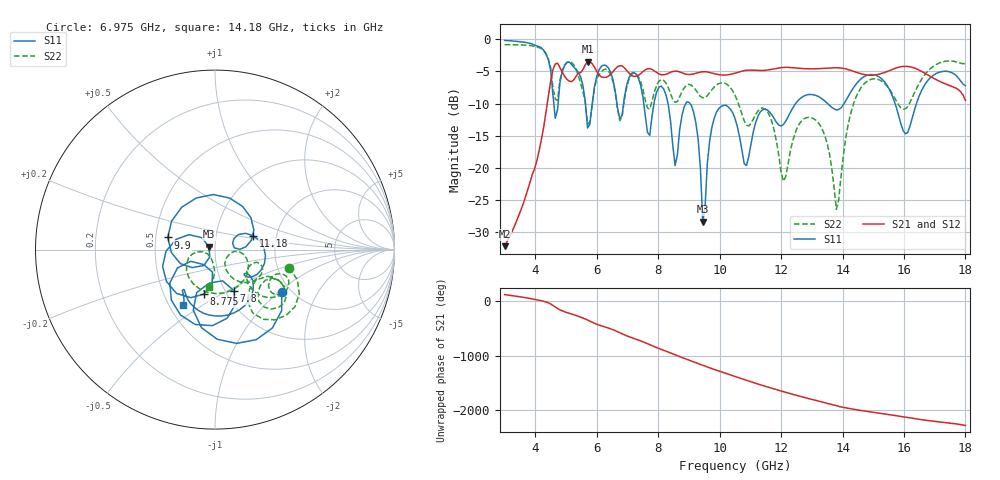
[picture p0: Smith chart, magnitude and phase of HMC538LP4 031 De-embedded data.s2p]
! Chelmsford, MA 01824
! http://www.hittite.com
! Tel: 978-250-3343
! Fax: 978-250-3373
! Device  :  HMC538LP4
! Description:  600 Analog Phase Shifter
! Frequency  :  6.0 GHz - 15.0 GHz
! Package  :  LP4  - 4x4 mm Quad Flatpack No-Lead (QFN) Plastic Package: 24 pin
! Ports  :  2 RF, 1 DC
!  Pin  3  = Rfin  = Port 1
!  Pin  16  = Rfout = Port 2
!  pin  21  = vCTL
! Voltages:  VCTL  = 0 to 5.0 Volts
! Currents :  Vb(V)  Vd(V)  Ib(mA)  Id(mA)
!  0.00  3.10  0.000000	0.467830
! Data:  The device was measured on evaluation board 111296-1.
!  Data was collected using a calibrated network analyzer.
!  The evaluation circuit board was modeled and simulated.This was use
!  to removed the evaluation board circuit from the measured data.
!  The reference plane is the center of the package pin.
! Misc:  Lot #
!Date Measured:  03 - 11 -2009
! Date:  03 - 17 -2009
! Note:
!  Hittite Microwave supplies this data as a sample of measured data at the
!  package pin for this package product.  Your particular data for this product
!  may vary.
!  Data was taken at 25 degrees C.
!  Hittite Microwave reserves the right to change this data at anytime.
# MHz S MA R 50
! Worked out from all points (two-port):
!   201 points, 3 GHz to 18 GHz, reference 50 ohm
!   highest |S21| = -3.51 dB at 5.7 GHz (marker M1); lowest = -32.2 dB at 3 GHz (marker M2)
!   |S21| within 3 dB of the highest: 4.5 GHz to 5.099 GHz (599.2 MHz wide, 12.5 % of centre); 5.203 GHz to 17.14 GHz (11.94 GHz wide, 107 % of centre)
!   lowest |S11| = -28.4 dB at 9.45 GHz (marker M3), VSWR 1.08, Z = 46.6 + j1.46 ohm
!   |S11| at or under -10 dB: 8.32 GHz to 8.9 GHz (579.6 MHz wide, 6.73 % of centre); 9.033 GHz to 12.48 GHz (3.444 GHz wide, 32 % of centre); 15.71 GHz to 16.41 GHz (698.2 MHz wide, 4.35 % of centre)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
!   |S22| runs from -26.4 to -0.9 dB; largest |S21 - S12| = 0.0044
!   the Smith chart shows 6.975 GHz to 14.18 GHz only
!   S11 on the Smith chart (normalised r, x): 6.975 GHz: 1.79, -1.05; 7.8 GHz: 1.10, -0.54; 8.775 GHz: 0.78, -0.42; 9.9 GHz: 0.58, +0.08; 11.18 GHz: 1.51, +0.25; 14.18 GHz: 0.59, -0.42
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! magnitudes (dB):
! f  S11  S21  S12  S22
! 3 GHz  -0.2  -32.2  -32.2  -0.9
! 4.275 GHz  -1.7  -13.6  -13.6  -1.8
! 4.65 GHz  -12.3  -3.8  -3.9  -9.3
! 5.55 GHz  -7.2  -4.7  -4.8  -8.1
! 5.7 GHz  -13.8  -3.5  -3.5  -13.2
! 6.15 GHz  -4.2  -5.9  -5.9  -5.1
! 6.975 GHz  -7.1  -4.9  -4.9  -7.4
! 7.8 GHz  -11.9  -4.7  -4.7  -9.6
! 8.025 GHz  -7.5  -5.4  -5.4  -6.5
! 8.55 GHz  -19.6  -5.0  -5.0  -9.8
! 8.775 GHz  -11.8  -5.2  -5.2  -8.1
! 9.225 GHz  -13.0  -5.3  -5.3  -7.9
! 9.45 GHz  -28.4  -5.1  -5.1  -9.1
! 9.9 GHz  -11.3  -5.5  -5.5  -7.1
! 10.5 GHz  -12.3  -5.3  -5.3  -8.7
! 11.18 GHz  -12.9  -4.8  -4.9  -11.7
! 12.07 GHz  -13.3  -4.4  -4.4  -22.1
! 13.05 GHz  -8.6  -4.6  -4.6  -12.3
! 13.8 GHz  -11.0  -4.4  -4.5  -26.4
! 14.18 GHz  -9.0  -4.7  -4.7  -13.5
! 15.53 GHz  -7.8  -4.9  -4.9  -7.8
! 18 GHz  -7.2  -9.5  -9.5  -3.8
